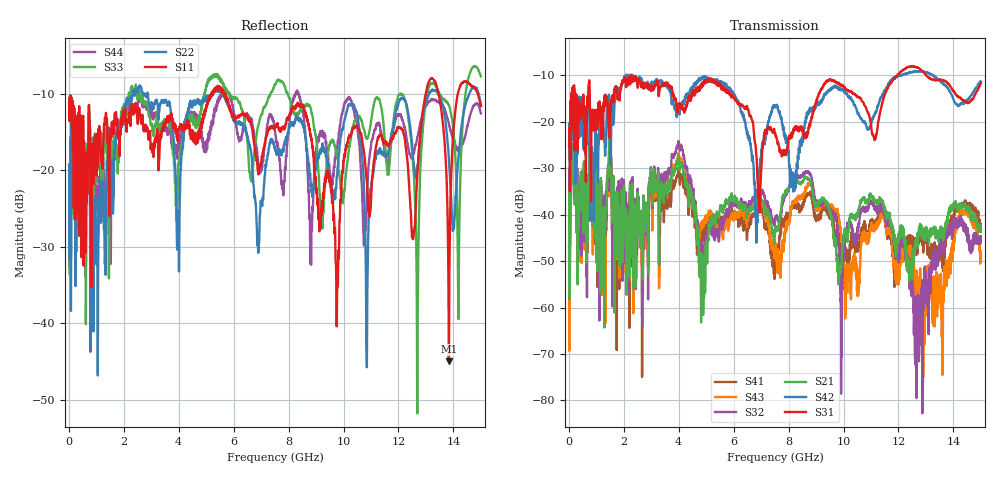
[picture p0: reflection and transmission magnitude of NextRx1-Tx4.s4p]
!  = SDD11
!  = SDD12
!  = SDC11
!  = SDC12
!  = SDD21
!  = SDD22
!  = SDC21
!  = SDC22
!  = SCD11
!  = SCD12
!  = SCC11
!  = SCC12
!  = SCD21
!  = SCD22
!  = SCC21
!  = SCC22
! FILE: N:\QM 2007\Prüfprotokolle\Highspeed\Konfektionierte Ltg\L45593-D106\D30\8216\0002\Next  Platine 2\NextRx1-Tx4.s4p
# MHz S DB R 50.00
! FREQ  S11  S12  S13  S14
!  S21  S22  S23  S24
!  S31  S32  S33  S34
!  S41  S42  S43  S44
!  DB  ANG  DB  ANG  DB  ANG  DB  ANG
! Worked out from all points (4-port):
!   2999 points, 10 MHz to 15 GHz, reference 50 ohm
!   strongest paths, dB at 10 MHz, 3.755 GHz, 7.505 GHz, 11.26 GHz, 15 GHz:
!     S31: -25.4, -12.7, -22.4, -20.3, -11.7
!     S42: -24.7, -15.8, -16.9, -16.7, -11.3
!     S21: -45.4, -30.0, -43.6, -37.4, -43.7
!     S32: -40.6, -27.0, -41.3, -39.2, -44.7
!     S43: -51.1, -29.2, -47.9, -42.4, -49.3
!     S41: -46.3, -32.4, -49.0, -40.8, -43.2
!   lowest |S11| = -44.9 dB at 13.84 GHz (marker M1), VSWR 1.01, Z = 50 - j0.566 ohm
!   |S11| at or under -10 dB: start of sweep to 5.185 GHz; 5.664 GHz to 12.99 GHz (7.331 GHz wide, 78.6 % of centre); 13.46 GHz to 14.16 GHz (703.5 MHz wide, 5.09 % of centre)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
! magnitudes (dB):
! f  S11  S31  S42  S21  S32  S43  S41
! 10 MHz  -11.3  -25.4  -24.7  -45.4  -40.6  -51.1  -46.3
! 145 MHz  -17.3  -17.6  -18.5  -25.5  -25.1  -25.4  -25.2
! 4.855 GHz  -13.5  -12.3  -10.5  -51.4  -45.9  -42.0  -44.5
! 8.675 GHz  -13.5  -23.1  -18.2  -32.2  -30.9  -34.2  -35.9
! 12.62 GHz  -25.3  -8.2  -9.1  -46.0  -65.5  -55.1  -46.4
! 13.84 GHz  -44.9  -11.9  -13.1  -39.3  -43.8  -51.9  -43.1
! 15 GHz  -11.6  -11.7  -11.3  -43.7  -44.7  -49.3  -43.2
